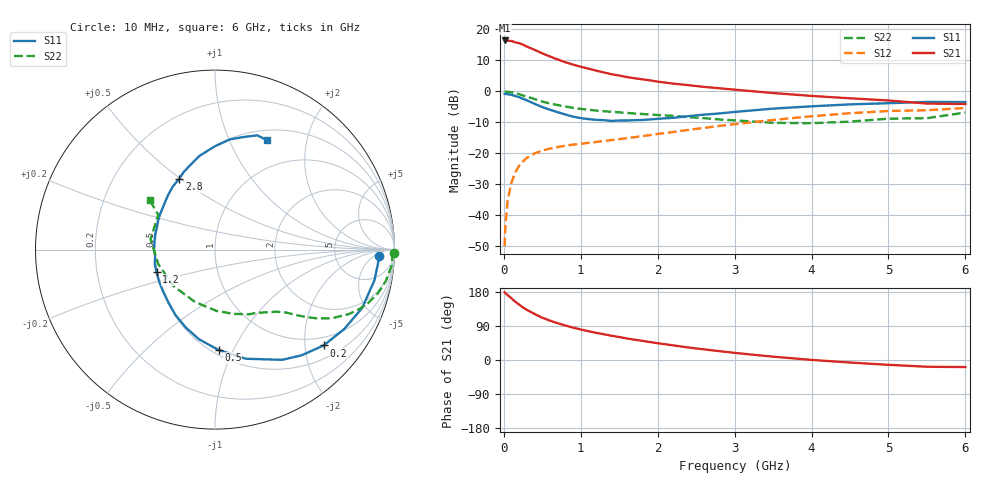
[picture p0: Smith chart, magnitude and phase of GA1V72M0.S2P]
! Infineon Technologies  Discrete & RF Semiconductors
! BF775
! Si NPN RF Bipolar Junction Transistor in SOT23
! VCE = 1.75 V  IC = 2 mA
! Common Emitter S-Parameters:  May  1996
# GHz  S  MA  R  50
!  f  S11  S21  S12  S22
! GHz  MAG  ANG  MAG  ANG  MAG  ANG  MAG  ANG
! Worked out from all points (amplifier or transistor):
!   36 points, 10 MHz to 6 GHz, reference 50 ohm
!   highest |S21| = 16.5 dB at 10 MHz (marker M1)
!   |S21| within 3 dB of that: start of sweep to 397 MHz
!   unconditionally stable (mu >= 1): 1.122 GHz to end of sweep
!   at 250 MHz: K = 0.29, MSG = 18.8 dB, |S12| = -22.5 dB
!   at 1.4 GHz: K = 1.13, MAG = 8.4 dB, |S12| = -15.7 dB
!   at 6 GHz: K = 1.03, MAG = -0.4 dB, |S12| = -5.3 dB
!   S11 on the Smith chart (normalised r, x): 10 MHz: 19, -8; 200 MHz: 0.79, -2.42; 500 MHz: 0.54, -0.88; 1.2 GHz: 0.50, -0.14; 2.8 GHz: 0.50, +0.49; 6 GHz: 0.62, +1.39
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0.01  0.9143 -2.1  6.65 178.6  0.0032 87.6  0.9975 -1.0
0.02  0.9122 -4.4  6.532 176.4  0.007 87.6  0.9889 -2.1
0.05  0.905 -10.8  6.596 171.2  0.0176 83.7  0.9878 -5.3
0.1  0.8819 -21.7  6.513 162.6  0.0343 78.2  0.9681 -10.4
0.15  0.845 -31.6  6.189 153.6  0.0499 71.9  0.9391 -15.1
0.2  0.8075 -41.4  6.001 145.9  0.0636 66.4  0.9034 -19.3
0.25  0.7609 -50.8  5.684 138.5  0.0749 61.8  0.8617 -23.1
0.3  0.7187 -58.7  5.282 132.2  0.0852 58.5  0.8254 -25.9
0.4  0.632 -74.2  4.691 121.4  0.1005 52.3  0.7534 -30.5
0.5  0.5594 -88.0  4.117 111.5  0.1112 47.8  0.687 -33.9
0.6  0.5076 -100.1  3.662 103.9  0.1201 45.0  0.6395 -36.1
0.8  0.4252 -121.3  2.959 91.0  0.1337 41.8  0.5722 -39.3
0.9  0.3926 -131.3  2.711 85.4  0.1388 41.3  0.5452 -40.6
1.1  0.3588 -150.2  2.335 76.0  0.1485 41.0  0.507 -43.4
1.2  0.3488 -159.1  2.169 71.6  0.1534 41.1  0.4927 -44.7
1.6  0.3404 172.0  1.704 56.7  0.1768 42.0  0.451 -50.8
2.2  0.3759 139.9  1.338 38.7  0.2219 43.0  0.4046 -63.3
2.8  0.4419 116.8  1.128 23.4  0.2783 41.0  0.3537 -81.0
3.5  0.5291 99.5  0.944 8.8  0.3475 34.9  0.3122 -111.1
4.5  0.6191 82.4  0.776 -6.7  0.4462 22.6  0.3261 -165.6
5.5  0.6786 69.7  0.638 -17.8  0.4982 7.4  0.3711 148.5
6  0.6752 64.5  0.628 -18.6  0.5426 3.2  0.4573 142.8
